(* Logix 5000 AddOnInstructionDefinition export AMCI_SV160E2_Hold; software revision 20.03 *)

ADD_ON_INSTRUCTION AMCI_SV160E2_Hold   (* revision 1.0, vendor AMCI *)
// Revision note:
// 8/2019 Version 0 Initial release of SV160E2 Add On Instructions.
// 3/17/20 Version 1 replaced the generic EDS file with a more complete V1.6 EDS file.
VAR_IN_OUT
   AMCI_SV160E2_OUTPUT_DATA : _000A:SV160E2_9125ACD4:O:0; {required}
END_VAR
VAR
   command_data_block : INT[10];
        [0]   // Command Bits MSW
        [1]   // Command Bits LSW
        [2]   // Upper Target Position
        [3]   // Lower Target Position
        [4]   // Upper Programmed Speed
        [5]   // Lower Programmed Speed
END_VAR

ROUTINE Logic   (* ladder *)
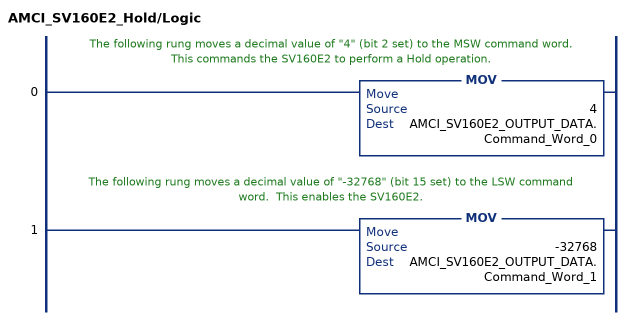
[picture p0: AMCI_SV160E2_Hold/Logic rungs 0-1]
   // The following rung moves a decimal value of "4" (bit 2 set) to the MSW command word.  This commands the SV160E2 to perform a Hold operation.
   0: MOV(4,AMCI_SV160E2_OUTPUT_DATA.Command_Word_0);
   // The following rung moves a decimal value of "-32768" (bit 15 set) to the LSW command word.  This enables the SV160E2.
   1: MOV(-32768,AMCI_SV160E2_OUTPUT_DATA.Command_Word_1);
END_ROUTINE
END_ADD_ON_INSTRUCTION
